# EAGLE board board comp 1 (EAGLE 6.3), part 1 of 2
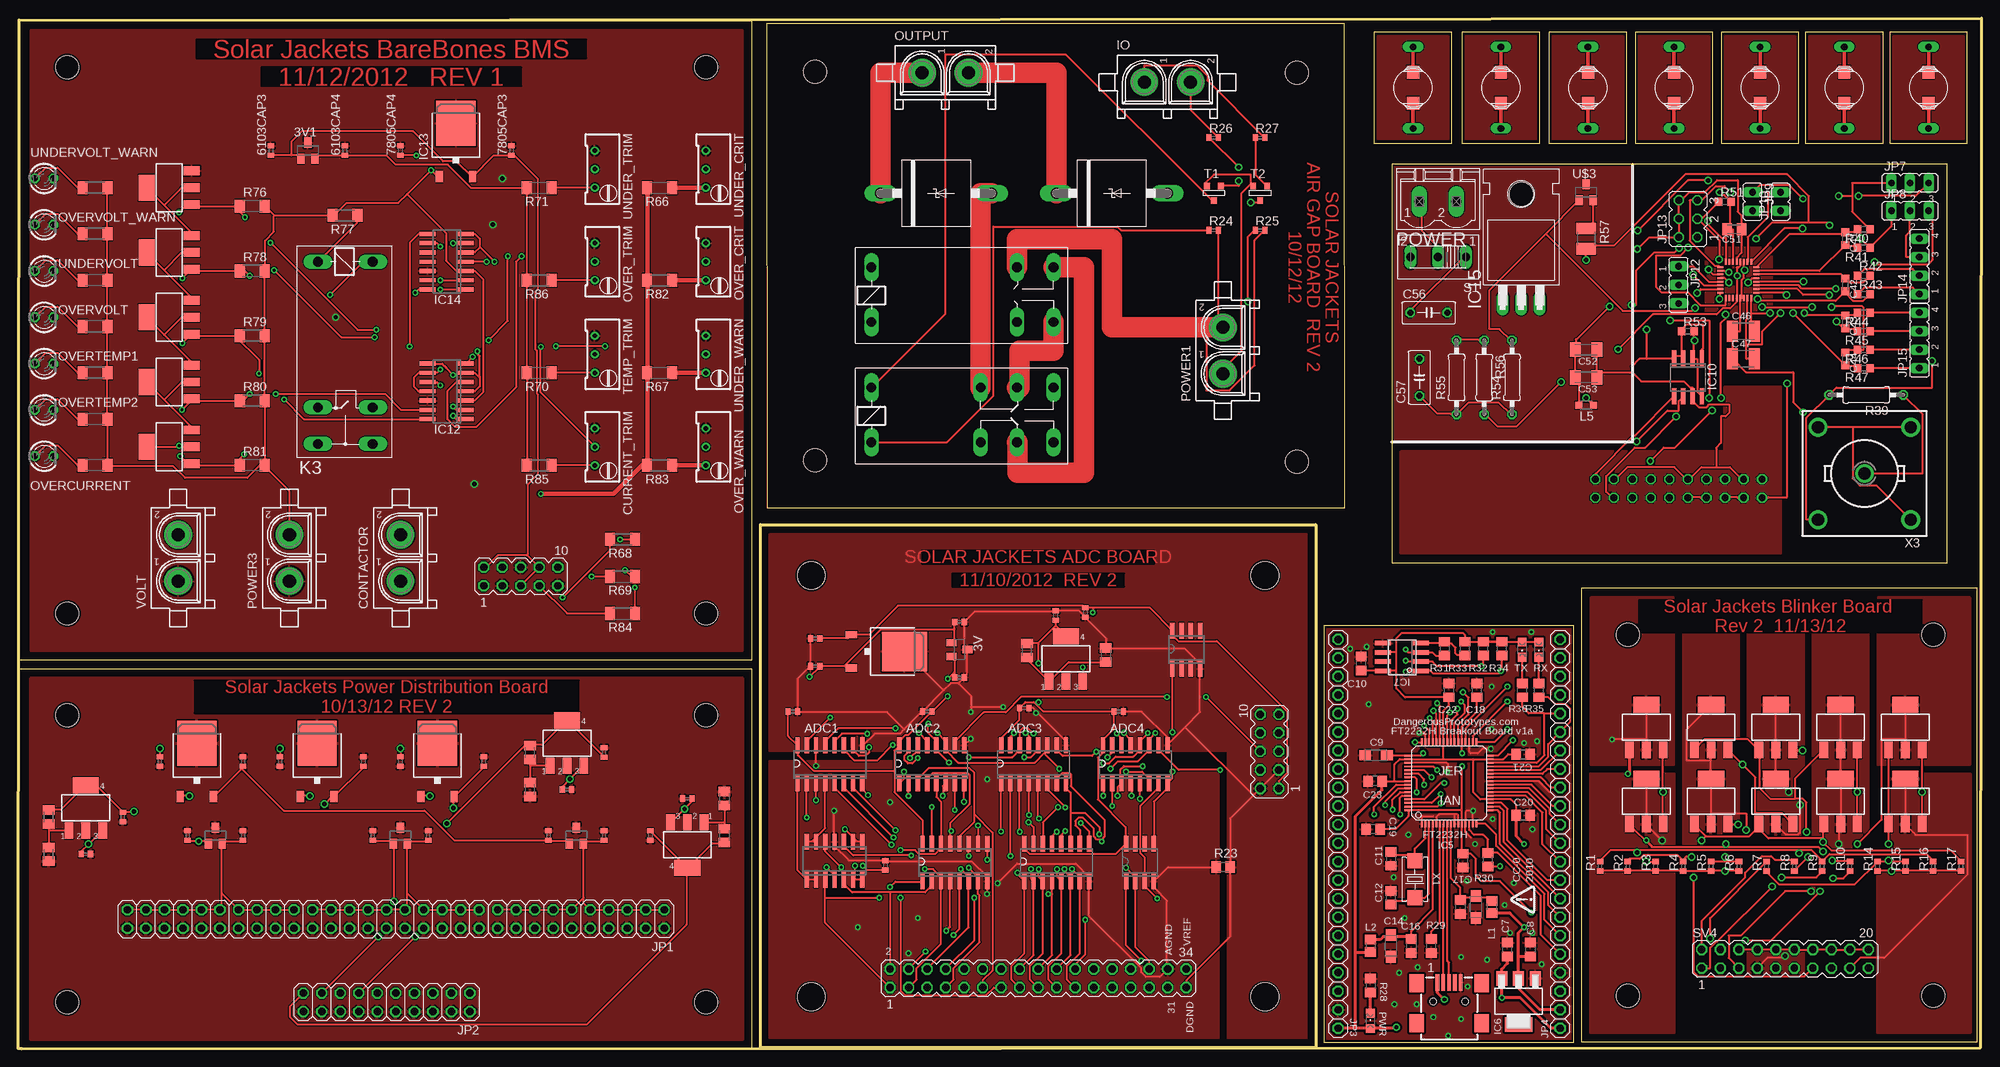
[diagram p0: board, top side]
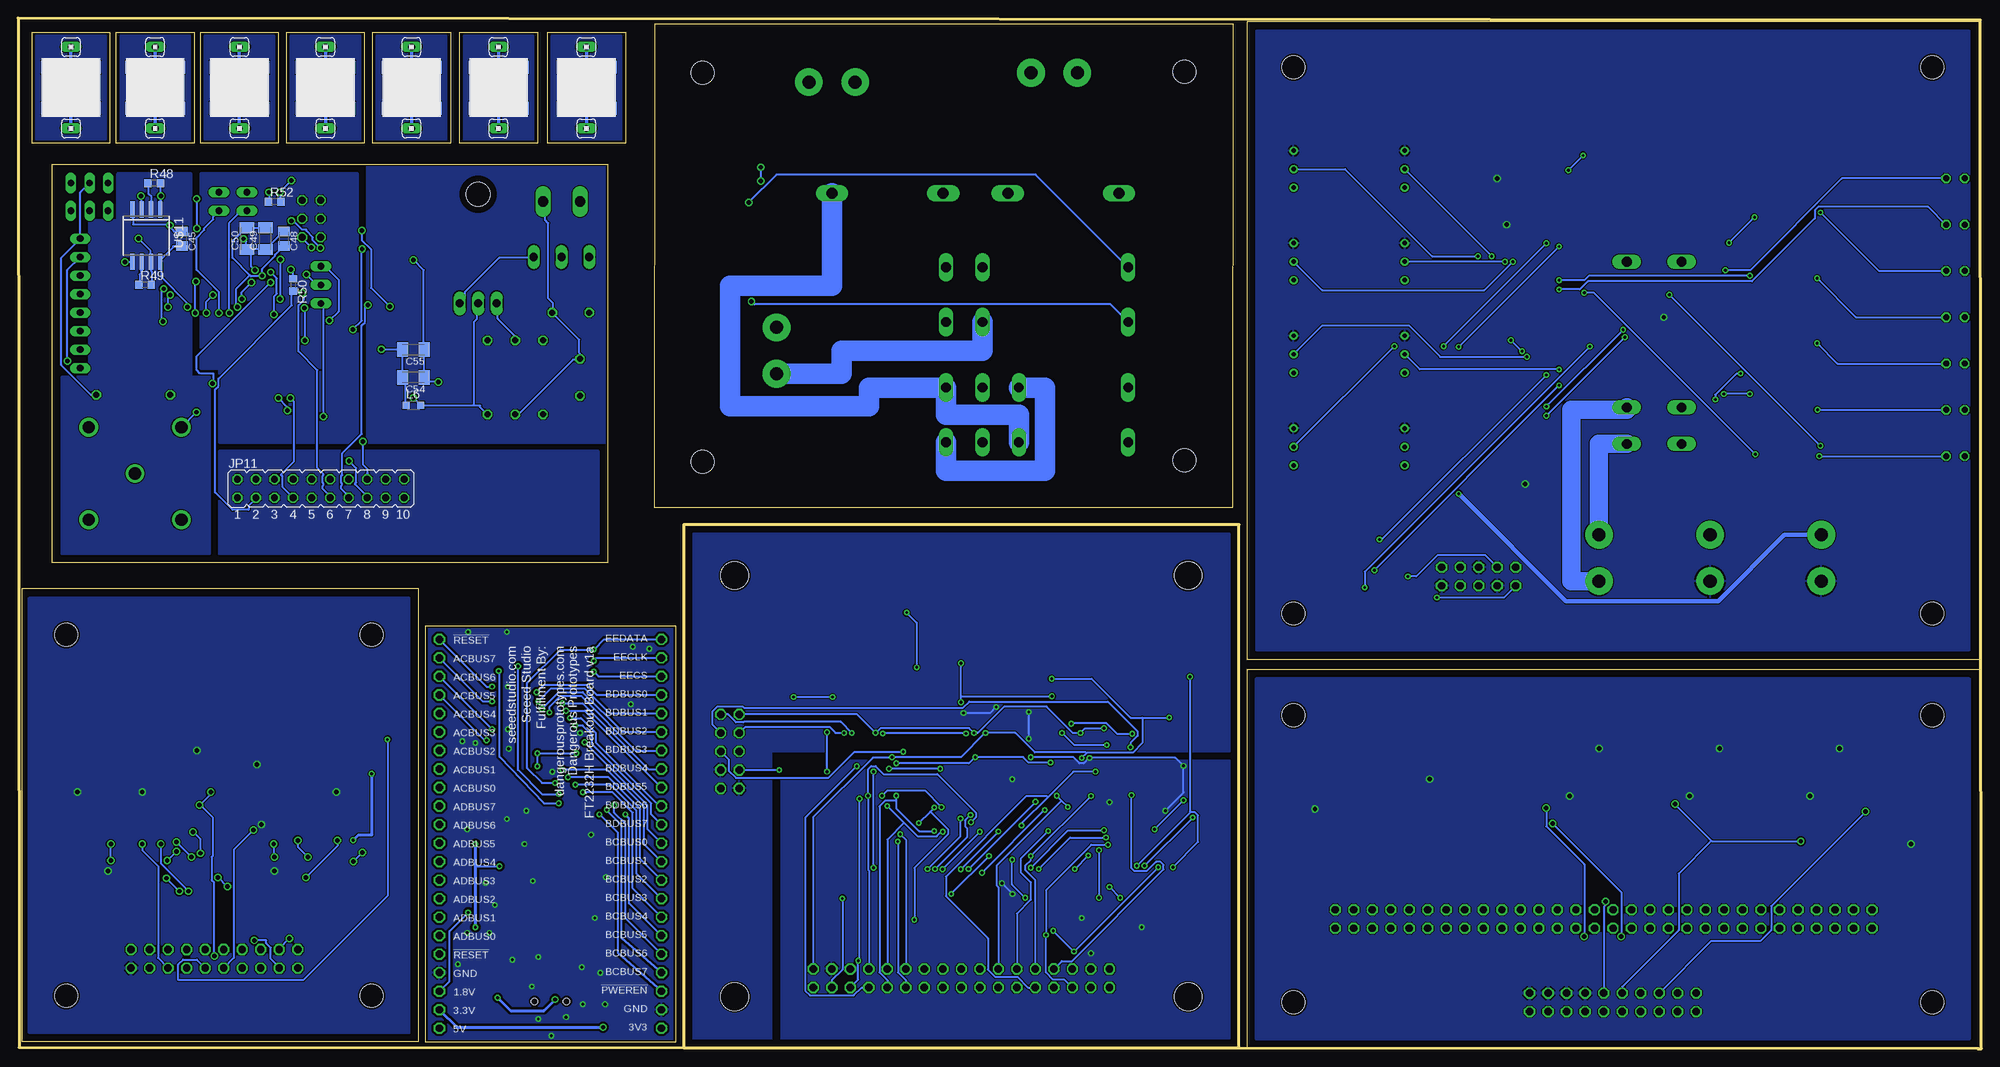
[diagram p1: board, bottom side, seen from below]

Size 269.37 x 141.35 mm. Coordinates in mm from the lower left corner, seen from the top.
Outline: 63 segments
Copper layers (1*16): Top 0.035mm / dielectric 1.5mm / Bottom 0.035mm
Design rules "default *": minimum track width 8mil, minimum drill 15mil, track to track 6mil, track to pad 6mil, pad to pad 6mil, via to via 6mil, smd to smd 6mil, copper to edge 10mil, drill to drill 8mil, minimum pad ring 10mil, minimum via ring 8mil, stop-mask expansion 4mil, vias tented up to drill 0mil, thermal gap 10mil
Holes 3.17 mm at 94.36,59.69 6.73,59.69 94.36,134.62 6.73,134.62 220.85,56.77 220.85,7.24 262.76,56.77 262.76,7.24 94.36,6.35 6.73,6.35 6.73,45.72 94.36,45.72 109.32,80.7 175.48,133.86 175.48,80.52 109.32,134.04
Holes 3.81 mm at 171.07,64.9 108.84,64.9 171.07,7.11 108.84,7.11

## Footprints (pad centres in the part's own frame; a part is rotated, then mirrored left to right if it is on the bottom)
SOT23 = smd 1 x 1.4: 1 -0.95,-1.1; 2 0.95,-1.1; 3 0,1.1
TO252 = smd 1 x 1.6: 1 -2.28,-4.8; 2 2.28,-4.8 | smd 5.4 x 6.2: 3 0,2.5
C0402 = smd 0.7 x 0.9: 1 -0.65,0; 2 0.65,0
SO16 = smd 0.6 x 2.2: 1 -4.445,-2.6; 2 -3.175,-2.6; 3 -1.905,-2.6; 4 -0.635,-2.6; 5 0.635,-2.6; 6 1.905,-2.6; 7 3.175,-2.6; 8 4.445,-2.6; 9 4.445,2.6; 10 3.175,2.6; 11 1.905,2.6; 12 0.635,2.6; 13 -0.635,2.6; 14 -1.905,2.6; 15 -3.175,2.6; 16 -4.445,2.6
SOT223 = smd 1.219 x 2.235: 1 -2.311,-3.099; 2 0,-3.099; 3 2.311,-3.099 | smd 3.6 x 2.2: 4 0,3.099
C805 = smd 1.3 x 1.5: 1 -0.95,0; 2 0.95,0
SMC_A = smd 1.6 x 1.4: + -1.5,0; - 1.5,0
C0603K = smd 1.05 x 1.08: 1 -0.875,0; 2 0.875,0
C0805K = smd 1.3 x 1.6: 1 -1,0; 2 1,0
C1210K = smd 1.5 x 2.9: 1 -1.5,0; 2 1.5,0
C1206K = smd 1.5 x 2: 1 -1.5,0; 2 1.5,0
C050-030X075 = drill 0.813 octagon: 1 -2.54,0; 2 2.54,0
CONN_USB_MINI-B = smd 2 x 2.5: BODY@1 -4.45,2.5; BODY@2 4.45,2.5; BODY@3 4.45,-3; BODY@4 -4.45,-3 | smd 0.5 x 2.3: D+ 0,2.6; D- -0.8,2.6; GND 1.6,2.6; ID 0.8,2.6; VUSB -1.6,2.6 | hole 0.9: -2.2,0; 2.2,0
350428-1 = drill 1.8 pad 3.81: 1 -3.175,0; 2 3.175,0
RTRIM64W = drill 0.61: 1 1.27,-2.54; 2 1.27,0; 3 1.27,2.54
P6T15 = drill 1.499 long: A 7.62,0; C -7.62,0
LQFP64 = smd 1 x 0.27: 1 -5.6,3.75; 2 -5.6,3.25; 3 -5.6,2.75; 4 -5.6,2.25; 5 -5.6,1.75; 6 -5.6,1.25; 7 -5.6,0.75; 8 -5.6,0.25; 9 -5.6,-0.25; 10 -5.6,-0.75; 11 -5.6,-1.25; 12 -5.6,-1.75; 13 -5.6,-2.25; 14 -5.6,-2.75; 15 -5.6,-3.25; 16 -5.6,-3.75; 33 5.6,-3.75; 34 5.6,-3.25; 35 5.6,-2.75; 36 5.6,-2.25; 37 5.6,-1.75; 38 5.6,-1.25; 39 5.6,-0.75; 40 5.6,-0.25; 41 5.6,0.25; 42 5.6,0.75; 43 5.6,1.25; 44 5.6,1.75; 45 5.6,2.25; 46 5.6,2.75; 47 5.6,3.25; 48 5.6,3.75 | smd 0.27 x 1: 17 -3.75,-5.6; 18 -3.25,-5.6; 19 -2.75,-5.6; 20 -2.25,-5.6; 21 -1.75,-5.6; 22 -1.25,-5.6; 23 -0.75,-5.6; 24 -0.25,-5.6; 25 0.25,-5.6; 26 0.75,-5.6; 27 1.25,-5.6; 28 1.75,-5.6; 29 2.25,-5.6; 30 2.75,-5.6; 31 3.25,-5.6; 32 3.75,-5.6; 49 3.75,5.6; 50 3.25,5.6; 51 2.75,5.6; 52 2.25,5.6; 53 1.75,5.6; 54 1.25,5.6; 55 0.75,5.6; 56 0.25,5.6; 57 -0.25,5.6; 58 -0.75,5.6; 59 -1.25,5.6; 60 -1.75,5.6; 61 -2.25,5.6; 62 -2.75,5.6; 63 -3.25,5.6; 64 -3.75,5.6
SOT223' = smd 1.5 x 2: 1 -2.3,-3.15; 2 0,-3.15; 3 2.3,-3.15 | smd 3.8 x 2: 4 0,3.15
SOIC8 = smd 0.6 x 2.2: 1 -1.905,-2.6; 2 -0.635,-2.6; 3 0.635,-2.6; 4 1.905,-2.6; 5 1.905,2.6; 6 0.635,2.6; 7 -0.635,2.6; 8 -1.905,2.6
SO-08 = smd 0.6 x 2.2: 1 -1.905,-2.6; 2 -0.635,-2.6; 3 0.635,-2.6; 4 1.905,-2.6; 5 1.905,2.6; 6 0.635,2.6; 7 -0.635,2.6; 8 -1.905,2.6
SO14 = smd 0.6 x 2.2: 1 -3.81,-2.6; 2 -2.54,-2.6; 3 -1.27,-2.6; 4 0,-2.6; 5 1.27,-2.6; 6 2.54,-2.6; 7 3.81,-2.6; 8 3.81,2.6; 9 2.54,2.6; 10 1.27,2.6; 11 0,2.6; 12 -1.27,2.6; 13 -2.54,2.6; 14 -3.81,2.6
TO220H = drill 1.118 long: 1 -2.54,-10.16; 2 0,-10.16; 3 2.54,-10.16 | hole 3.302: 0,4.826
2X30 = drill 1.016 octagon: 1 -38.1,-1.27; 2 -38.1,1.27; 3 -35.56,-1.27; 4 -35.56,1.27; 5 -33.02,-1.27; 6 -33.02,1.27; 7 -30.48,-1.27; 8 -30.48,1.27; 9 -27.94,-1.27; 10 -27.94,1.27; 11 -25.4,-1.27; 12 -25.4,1.27; 13 -22.86,-1.27; 14 -22.86,1.27; 15 -20.32,-1.27; 16 -20.32,1.27; 17 -17.78,-1.27; 18 -17.78,1.27; 19 -15.24,-1.27; 20 -15.24,1.27; 21 -12.7,-1.27; 22 -12.7,1.27; 23 -10.16,-1.27; 24 -10.16,1.27; 25 -7.62,-1.27; 26 -7.62,1.27; 27 -5.08,-1.27; 28 -5.08,1.27; 29 -2.54,-1.27; 30 -2.54,1.27; 31 0,-1.27; 32 0,1.27; 33 2.54,-1.27; 34 2.54,1.27; 35 5.08,-1.27; 36 5.08,1.27; 37 7.62,-1.27; 38 7.62,1.27; 39 10.16,-1.27; 40 10.16,1.27; 41 12.7,-1.27; 42 12.7,1.27; 43 15.24,-1.27; 44 15.24,1.27; 45 17.78,-1.27; 46 17.78,1.27; 47 20.32,-1.27; 48 20.32,1.27; 49 22.86,-1.27; 50 22.86,1.27; 51 25.4,-1.27; 52 25.4,1.27; 53 27.94,-1.27; 54 27.94,1.27; 55 30.48,-1.27; 56 30.48,1.27; 57 33.02,-1.27; 58 33.02,1.27; 59 35.56,-1.27; 60 35.56,1.27
2X10 = drill 1.016 octagon: 1 -11.43,-1.27; 2 -11.43,1.27; 3 -8.89,-1.27; 4 -8.89,1.27; 5 -6.35,-1.27; 6 -6.35,1.27; 7 -3.81,-1.27; 8 -3.81,1.27; 9 -1.27,-1.27; 10 -1.27,1.27; 11 1.27,-1.27; 12 1.27,1.27; 13 3.81,-1.27; 14 3.81,1.27; 15 6.35,-1.27; 16 6.35,1.27; 17 8.89,-1.27; 18 8.89,1.27; 19 11.43,-1.27; 20 11.43,1.27
1X22 = drill 1.016 octagon: 1 -26.67,0; 2 -24.13,0; 3 -21.59,0; 4 -19.05,0; 5 -16.51,0; 6 -13.97,0; 7 -11.43,0; 8 -8.89,0; 9 -6.35,0; 10 -3.81,0; 11 -1.27,0; 12 1.27,0; 13 3.81,0; 14 6.35,0; 15 8.89,0; 16 11.43,0; 17 13.97,0; 18 16.51,0; 19 19.05,0; 20 21.59,0; 21 24.13,0; 22 26.67,0
JP2 = drill 0.914 long: 1 -2.54,0; 2 0,0; 3 2.54,0
JP1 = drill 0.914 long: 1 0,-1.27; 2 0,1.27
JP10Q = drill 0.914 octagon: 1 -11.43,-1.27; 2 -11.43,1.27; 3 -8.89,-1.27; 4 -8.89,1.27; 5 -6.35,-1.27; 6 -6.35,1.27; 7 -3.81,-1.27; 8 -3.81,1.27; 9 -1.27,-1.27; 10 -1.27,1.27; 11 1.27,-1.27; 12 1.27,1.27; 13 3.81,-1.27; 14 3.81,1.27; 15 6.35,-1.27; 16 6.35,1.27; 17 8.89,-1.27; 18 8.89,1.27; 19 11.43,-1.27; 20 11.43,1.27
JP3Q = drill 0.914 octagon: 1 -2.54,-1.27; 2 -2.54,1.27; 3 0,-1.27; 4 0,1.27; 5 2.54,-1.27; 6 2.54,1.27
JP4 = drill 0.914 long: 1 -3.81,0; 2 -1.27,0; 3 1.27,0; 4 3.81,0
G2R2 = drill 1.321 long: 1 -2.54,-3.683; 2 -2.54,3.81; O1 12.471,3.81; O2 12.471,-3.683; P1 17.45,3.81; P2 17.45,-3.683; S1 22.454,3.81; S2 22.454,-3.683
G2R2A = drill 1.321 long: 1 -2.54,-3.683; 2 -2.54,3.81; P1 17.45,3.81; P2 17.45,-3.683; S1 22.454,3.81; S2 22.454,-3.683
G2REA = drill 1.321 long: 1 -2.54,-3.683; 2 -2.54,3.81; P 17.45,-3.683; P@ 17.45,3.81; S 22.454,-3.683; S@ 22.454,3.81
FB805 = smd 1.3 x 1.5: 1 -0.85,0; 2 0.85,0
L2012C = smd 1 x 1: 1 -1,0; 2 1,0
LQH55PN220MR0L = smd 1.8 x 1.7: P$1 -2.135,0; P$2 2.135,0
NRS8040T0R9NJGJ = smd 8.2 x 1.8: P$1 0,2.8; P$2 0,-2.8
LED3MM = drill 0.813 octagon: A -1.27,0; K 1.27,0
MSTBV2 = drill 1.397 long: 1 -2.54,0; 2 2.54,0
LED-805 = smd 1.2 x 1.2: A 0,-1.05; C 0,1.05
R0402 = smd 0.7 x 0.9: 1 -0.65,0; 2 0.65,0
M0805 = smd 1.3 x 1.6: 1 -0.95,0; 2 0.95,0
R805 = smd 1.3 x 1.5: 1 -0.95,0; 2 0.95,0
0207/10 = drill 0.813 octagon: 1 -5.08,0; 2 5.08,0
R0603 = smd 1 x 1.1: 1 -0.85,0; 2 0.85,0
R3225 = smd 1.6 x 2.7: 1 -1.4,0; 2 1.4,0
M1406 = smd 1.4 x 1.8: 1 -1.7,0; 2 1.7,0
255SB = drill 1.118 long: 1 -3.81,0; 2 0,0; 3 3.81,0
MA17-2 = drill 1.016 octagon: 1 -20.32,-1.27; 2 -20.32,1.27; 3 -17.78,-1.27; 4 -17.78,1.27; 5 -15.24,-1.27; 6 -15.24,1.27; 7 -12.7,-1.27; 8 -12.7,1.27; 9 -10.16,-1.27; 10 -10.16,1.27; 11 -7.62,-1.27; 12 -7.62,1.27; 13 -5.08,-1.27; 14 -5.08,1.27; 15 -2.54,-1.27; 16 -2.54,1.27; 17 0,-1.27; 18 0,1.27; 19 2.54,-1.27; 20 2.54,1.27; 21 5.08,-1.27; 22 5.08,1.27; 23 7.62,-1.27; 24 7.62,1.27; 25 10.16,-1.27; 26 10.16,1.27; 27 12.7,-1.27; 28 12.7,1.27; 29 15.24,-1.27; 30 15.24,1.27; 31 17.78,-1.27; 32 17.78,1.27; 33 20.32,-1.27; 34 20.32,1.27
MA05-2 = drill 1.016 octagon: 1 -5.08,-1.27; 2 -5.08,1.27; 3 -2.54,-1.27; 4 -2.54,1.27; 5 0,-1.27; 6 0,1.27; 7 2.54,-1.27; 8 2.54,1.27; 9 5.08,-1.27; 10 5.08,1.27
MA10-2 = drill 1.016 octagon: 1 -11.43,-1.27; 2 -11.43,1.27; 3 -8.89,-1.27; 4 -8.89,1.27; 5 -6.35,-1.27; 6 -6.35,1.27; 7 -3.81,-1.27; 8 -3.81,1.27; 9 -1.27,-1.27; 10 -1.27,1.27; 11 1.27,-1.27; 12 1.27,1.27; 13 3.81,-1.27; 14 3.81,1.27; 15 6.35,-1.27; 16 6.35,1.27; 17 8.89,-1.27; 18 8.89,1.27; 19 11.43,-1.27; 20 11.43,1.27
SOT-23 = smd 0.787 x 0.889: 1 0.025,-1.016; 2 -0.94,1.016; 3 0.991,1.016
ADS8363 = smd 0.28 x 0.85: P$1_ 0.725,0.725; P$2_ 1.225,0.725; P$3_ 1.725,0.725; P$4_ 2.225,0.725; P$5_ 2.725,0.725; P$6_ 3.225,0.725; P$7_ 3.725,0.725; P$8_ 4.225,0.725; P$17_ 4.225,-4.225; P$18_ 3.725,-4.225; P$19_ 3.225,-4.225; P$20_ 2.725,-4.225; P$21_ 2.225,-4.225; P$22_ 1.725,-4.225; P$23_ 1.225,-4.225; P$24_ 0.725,-4.225 | smd 0.85 x 0.28: P$9_ 4.95,0; P$10_ 4.95,-0.5; P$11_ 4.95,-1; P$12_ 4.95,-1.5; P$13_ 4.95,-2; P$14_ 4.95,-2.5; P$15_ 4.95,-3; P$16_ 4.95,-3.5; P$25_ 0,-3.5; P$26_ 0,-3; P$27_ 0,-2.5; P$28_ 0,-2; P$29_ 0,-1.5; P$30_ 0,-1; P$31_ 0,-0.5; P$32_ 0,0
SINGLE_HEADER = drill 0.914 long: P$1 0,0
SOP-08 = smd 0.6 x 2.2: 1 -1.905,-3.6; 2 -0.635,-3.6; 3 0.635,-3.6; 4 1.905,-3.6; 5 1.905,3.575; 6 0.635,3.575; 7 -0.635,3.575; 8 -1.905,3.575
4X6 = smd 2.032 x 2.032: 1 -2.54,0; 2 2.54,0
B35N57 = drill 1.7: 1 0,0; 2 6.35,6.35; 3 -6.35,6.35; 4 -6.35,-6.35; 5 6.35,-6.35

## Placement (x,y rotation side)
3V  MAX6103  [SOT23]  129.16,54.74 270 top
3V1  MAX6103  [SOT23]  39.75,123.19 0 top
3V2  MAX6103  [SOT23]  76.58,29.21 0 top
3V3  MAX6103  [SOT23]  52.45,29.21 0 top
3V4  MAX6103  [SOT23]  27.05,29.21 0 top
5V  LM7805TV  [TO252]  119.13,54.48 270 top
317CAP1  .33uF  [C0402]  146.43,59.82 270 top
317CAP2  1uF  [C0402]  142.37,59.44 90 top
317CAP3  .33uF  [C0402]  9.27,26.67 0 top
317CAP4  1uF  [C0402]  14.35,31.75 270 top
317CAP5  .33uF  [C0402]  75.31,35.56 0 top
317CAP6  1uF  [C0402]  80.39,40.64 90 top
317CAP7  .33uF  [C0402]  91.82,34.29 180 top
317CAP8  1uF  [C0402]  86.74,29.21 270 top
6103CAP1  1uF  [C0402]  129.16,58.55 0 top
6103CAP2  1uF  [C0402]  129.16,50.93 0 top
6103CAP3  1uF  [C0402]  34.67,123.19 90 top
6103CAP4  1uF  [C0402]  44.83,123.19 90 top
6103CAP5  1uF  [C0402]  72.77,29.21 90 top
6103CAP6  1uF  [C0402]  80.39,29.21 90 top
6103CAP7  1uF  [C0402]  48.64,29.21 90 top
6103CAP8  1uF  [C0402]  56.26,29.21 90 top
6103CAP9  1uF  [C0402]  23.24,29.21 90 top
6103CAP10  1uF  [C0402]  30.86,29.21 90 top
6484CAP1  .1uF  [C0402]  119,25.15 90 top
7805CAP1  .33uF  [C0402]  109.35,56.26 180 top
7805CAP2  1uF  [C0402]  109.35,52.45 180 top
7805CAP3  1uF  [C0402]  67.69,123.19 90 top
7805CAP4  1uF  [C0402]  52.45,123.19 90 top
ADC1  MCP-3008  [SO16]  111.38,38.99 0 top
ADC2  MCP-3008  [SO16]  125.35,38.99 0 top
ADC3  MCP-3008  [SO16]  139.32,38.99 0 top
ADC4  MCP-3008  [SO16]  153.29,38.99 0 top
ADC_CAP1  .1uF  [C0402]  106.3,46.23 0 top
ADC_CAP2  .1uF  [C0402]  124.71,46.23 180 top
ADC_CAP3  .1uF  [C0402]  138.05,46.74 0 top
ADC_CAP4  .1uF  [C0402]  151,46.23 0 top
BLINKER-L1  N-HEXFET-2D_SOT232-  [SOT223]  223.39,44.07 0 top
BLINKER-L2  N-HEXFET-2D_SOT232-  [SOT223]  223.39,33.91 0 top
BLINKER-R1  N-HEXFET-2D_SOT232-  [SOT223]  258.95,44.07 0 top
BLINKER-R2  N-HEXFET-2D_SOT232-  [SOT223]  258.95,33.91 0 top
BRAKE-C1  N-HEXFET-2D_SOT232-  [SOT223]  241.17,44.07 0 top
BRAKE-C2  N-HEXFET-2D_SOT232-  [SOT223]  241.17,33.91 0 top
BRAKE-L1  N-HEXFET-2D_SOT232-  [SOT223]  232.28,44.07 0 top
BRAKE-L2  N-HEXFET-2D_SOT232-  [SOT223]  232.28,33.91 0 top
BRAKE-R1  N-HEXFET-2D_SOT232-  [SOT223]  250.06,44.07 0 top
BRAKE-R2  N-HEXFET-2D_SOT232-  [SOT223]  250.06,33.91 0 top
C1  1uF  [C0402]  19.43,39.37 270 top
C2  1uF  [C0402]  30.86,39.37 90 top
C3  1uF  [C0402]  35.94,39.37 270 top
C4  1uF  [C0402]  47.37,39.37 90 top
C5  1uF  [C0402]  52.45,39.37 270 top
C6  1uF  [C0402]  63.88,39.37 90 top
C7  0.1uF  [C805]  204.34,13.59 90 top
C8  0.1uF  [C805]  207.52,13.59 90 top
C9  3.3uF  [SMC_A]  186.31,40.26 180 top
C10  0.1uF  [C805]  184.28,52.83 90 top
C11  27pF  [C805]  188.34,26.04 270 top
C12  27pF  [C805]  188.34,20.7 90 top
C13  4.7uF  [SMC_A]  200.03,19.43 270 top
C14  4.7uF  [SMC_A]  188.34,14.1 270 top
C15  0.1uF  [C805]  197.87,19.43 270 top
C16  0.1uF  [C805]  191.13,14.1 270 top
C17  0.1uF  [C805]  198.25,25.78 270 top
C18  0.1uF  [C805]  200.15,49.15 90 top
C19  0.1uF  [C805]  185.93,30.1 180 top
C20  0.1uF  [C805]  206.5,32 0 top
C21  0.1uF  [C805]  206.5,40.39 0 top
C22  0.1uF  [C805]  196.34,49.15 90 top
C23  0.1uF  [C805]  186.18,36.7 180 top
C41  3900pF  [C0603K]  250.7,111.12 270 top
C42  3900pF  [C0603K]  250.7,104.78 270 top
C43  3900pF  [C0603K]  250.7,99.69 270 top
C44  3900pF  [C0603K]  250.7,94.61 270 top
C45  1uF  [C0805K]  246.89,111.12 270 bottom
C46  10uF  [C1210K]  236.73,98.42 0 top
C47  10uF  [C1210K]  236.73,94.61 0 top
C48  1uF  [C0805K]  232.92,111.12 270 bottom
C49  0.1uF  [C1206K]  235.46,111.12 90 bottom
C50  0.1uF  [C1206K]  238,111.12 90 bottom
C51  1uF  [C0805K]  235.46,112.39 180 top
C52  0.1uF  [C1206K]  215.14,95.89 180 top
C53  0.1uF  [C1206K]  215.14,92.08 180 top
C54  0.1uF  [C1206K]  215.14,92.08 180 bottom
C55  0.1uF  [C1206K]  215.14,95.89 180 bottom
C56  [C050-030X075]  193.55,100.97 0 top
C57  [C050-030X075]  192.28,92.08 90 top
CONN1  CONN_USB  [CONN_USB_MINI-B]  196.34,6.48 0 top
CONTACTOR  350428-1  [350428-1]  52.45,67.31 90 top
CURRENT_TRIM  1k  [RTRIM64W]  80.39,82.55 180 top
D1  5KPXX  [P6T15]  125.95,117.35 0 top
D2  5KPXX  [P6T15]  150.08,117.35 0 top
IC1  LM317  [SOT223]  75.31,41.91 0 top
IC2  LM317  [SOT223]  9.27,33.02 0 top
IC3  LM317  [SOT223]  91.82,27.94 180 top
IC4  LM317  [SOT223]  143.76,53.47 0 top
IC5  FT2232H  [LQFP64]  196.34,36.45 90 top
IC6  [SOT223']  205.87,6.48 180 top
IC7  93C46  [SOIC8]  189.87,53.72 90 top
IC10  24LC256T  [SO-08]  229.11,92.08 180 top
IC12  LM339D  [SO14]  58.8,90.17 90 top
IC13  7805DT  [TO252]  60.07,124.46 0 top
IC14  LM339D  [SO14]  58.8,107.95 90 top
IC15  317T  [TO220H]  206.25,112.39 0 top
IO  350428-1  [350428-1]  157.7,132.59 0 top
JP1  [2X30]  50.55,17.78 180 top
JP2  [2X10]  50.55,6.35 180 top
JP3  [1X22]  181.1,29.46 90 top
JP4  [1X22]  211.58,29.46 90 top
JP7  [JP2]  259.59,118.75 0 top
JP8  [JP2]  259.59,114.94 0 top
JP9  [JP1]  238,116.2 180 top
JP10  [JP1]  241.81,116.2 0 top
JP11  [JP10Q]  227.84,76.83 0 bottom
JP12  [JP2]  227.84,104.78 270 top
JP13  [JP3Q]  229.13,113.84 90 top
JP14  [JP4]  260.86,107.31 90 top
JP15  [JP4]  260.86,97.16 90 top
K1  G2R2  [G2R2]  119.6,86.87 0 top
K2  G2R2A  [G2R2A]  119.6,103.38 0 top
K3  G2REA  [G2REA]  44.83,105.41 270 top
L1  [FB805]  202.18,19.43 270 top
L2  [FB805]  185.55,14.1 270 top
L5  [L2012C]  215.14,88.27 180 top
L6  [L2012C]  215.14,88.27 0 bottom
LMC6484_1  LMC6484  [SO14]  112.01,25.78 0 top
NEWBATT  LQH55PN220MR0L  [LQH55PN220MR0L]  191.39,131.83 270 top
NEWBATT1  LQH55PN220MR0L  [LQH55PN220MR0L]  203.45,131.83 270 top
NEWBATT2  LQH55PN220MR0L  [LQH55PN220MR0L]  215.39,131.83 270 top
NEWBATT3  LQH55PN220MR0L  [LQH55PN220MR0L]  227.2,131.83 270 top
NEWBATT4  LQH55PN220MR0L  [LQH55PN220MR0L]  239.01,131.83 270 top
NEWBATT5  LQH55PN220MR0L  [LQH55PN220MR0L]  250.57,131.83 270 top
NEWBATT6  LQH55PN220MR0L  [LQH55PN220MR0L]  262.13,131.83 270 top
OLDBATT  NRS8040T0R9NJGJ  [NRS8040T0R9NJGJ]  191.39,131.83 0 bottom
OLDBATT1  NRS8040T0R9NJGJ  [NRS8040T0R9NJGJ]  203.45,131.83 0 bottom
OLDBATT2  NRS8040T0R9NJGJ  [NRS8040T0R9NJGJ]  215.39,131.83 0 bottom
OLDBATT3  NRS8040T0R9NJGJ  [NRS8040T0R9NJGJ]  227.2,131.83 0 bottom
OLDBATT4  NRS8040T0R9NJGJ  [NRS8040T0R9NJGJ]  239.01,131.83 0 bottom
OLDBATT5  NRS8040T0R9NJGJ  [NRS8040T0R9NJGJ]  250.57,131.83 0 bottom
OLDBATT6  NRS8040T0R9NJGJ  [NRS8040T0R9NJGJ]  262.13,131.83 0 bottom
OUTPUT  350428-1  [350428-1]  127.22,133.86 0 top
OVER_CRIT  10k  [RTRIM64W]  95.63,107.95 180 top
OVER_TRIM  1k  [RTRIM64W]  80.39,107.95 180 top
OVER_WARN  10K  [RTRIM64W]  95.63,82.55 180 top
OVERCURRENT  TLLG4400  [LED3MM]  3.56,81.28 0 top
OVERCURRENT_FET  N-HEXFET-2D_SOT232-  [SOT223]  20.7,82.55 90 top
OVERTEMP1  TLLG4400  [LED3MM]  3.56,93.98 0 top
OVERTEMP1_FET  N-HEXFET-2D_SOT232-  [SOT223]  20.7,100.33 90 top
OVERTEMP2  TLLG4400  [LED3MM]  3.56,87.63 0 top
OVERTEMP2_FET  N-HEXFET-2D_SOT232-  [SOT223]  20.7,91.44 90 top
OVERVOLT  TLLG4400  [LED3MM]  3.56,100.33 0 top
OVERVOLT_FET  N-HEXFET-2D_SOT232-  [SOT223]  20.7,109.22 90 top
OVERVOLT_WARN  TLLG4400  [LED3MM]  3.56,113.03 0 top
POWER  MSTBV2  [MSTBV2]  194.82,116.2 0 top
POWER1  350428-1  [350428-1]  165.32,95.76 90 top
POWER3  350428-1  [350428-1]  37.21,67.31 90 top
PWR  [LED-805]  185.55,3.81 0 top
PWR_1  7805DT  [TO252]  24.51,39.37 0 top
PWR_2  7805DT  [TO252]  41.02,39.37 0 top
PWR_3  7805DT  [TO252]  57.53,39.37 0 top
R1  1k  [R0402]  217.04,25.02 90 top
R2  1k  [R0402]  220.85,25.02 90 top
R3  1k  [R0402]  224.66,25.02 90 top
R4  1k  [R0402]  228.47,25.02 90 top
R5  1k  [R0402]  232.28,25.02 90 top
R6  1k  [R0402]  236.09,25.02 90 top
R7  1K  [R0402]  239.9,25.02 90 top
R8  1K  [R0402]  243.71,25.02 90 top
R9  1K  [R0402]  247.52,25.02 90 top
R10  1K  [R0402]  251.33,25.02 90 top
R11  220  [M0805]  4.19,31.75 270 top
R12  361  [M0805]  4.19,26.67 270 top
R13  220  [M0805]  70.23,40.64 270 top
R14  1k  [R0402]  255.14,25.02 90 top
R15  1k  [R0402]  258.95,25.02 90 top
R16  1k  [R0402]  262.76,25.02 90 top
R17  1k  [R0402]  266.57,25.02 90 top
R18  361  [M0805]  70.23,35.56 270 top
R19  220  [M0805]  96.9,29.21 90 top
R20  361  [M0805]  96.9,34.29 90 top
R21  220  [M0805]  138.43,54.61 270 top
R22  361  [M0805]  149.22,53.98 90 top
R23  0  [M0805]  165.35,24.89 0 top
R24  1k  [R0402]  164.05,112.27 0 top
R25  1k  [R0402]  170.4,112.27 0 top
R26  1k  [R0402]  164.05,124.97 0 top
R27  1k  [R0402]  170.4,124.97 0 top
R28  470  [R805]  185.55,8.64 270 top
R29  12k 1%  [R805]  193.93,14.1 90 top
R30  10k  [R805]  201.68,25.91 90 top
R31  2.2k  [R805]  195.71,54.86 270 top
R32  10k  [R805]  201.04,54.86 90 top
R33  10k  [R805]  198.5,54.86 90 top
R34  10k  [R805]  203.58,54.86 90 top
R35  470  [R805]  208.66,49.15 90 top
R36  470  [R805]  206.38,49.15 90 top
R39  1M  [0207/10]  253.57,89.69 180 top
R40  49.9  [R0603]  253.24,112.39 180 top
R41  49.9  [R0603]  253.24,109.86 180 top
R42  49.9  [R0603]  253.24,106.05 0 top
R43  49.9  [R0603]  253.24,103.5 0 top
R44  49.9  [R0603]  253.24,100.97 180 top
R45  49.9  [R0603]  253.24,98.42 180 top
R46  49.9  [R0603]  253.24,95.89 180 top
R47  49.9  [R0603]  253.24,93.34 180 top
R48  49.9  [R0603]  250.7,118.75 0 bottom
R49  49.9  [R0603]  251.97,104.78 0 bottom
R50  33  [R0603]  231.65,104.78 270 bottom
R51  10K  [R0603]  234.19,116.2 0 top
R52  10K  [R0603]  234.19,116.2 0 bottom
R53  33  [R0603]  229.11,98.42 0 top
R54  150  [0207/10]  204.98,92.08 90 top
R55  240  [0207/10]  197.36,92.08 90 top
R56  725  [0207/10]  201.17,92.08 270 top
R57  0  [R3225]  215.14,111.12 270 top
R66  100k  [M1406]  88.01,118.11 180 top
R67  100k  [M1406]  88.01,92.71 180 top
R68  100  [M1406]  82.93,69.85 180 top
R69  100  [M1406]  82.93,64.77 180 top
R70  100  [M1406]  71.5,92.71 180 top
R71  100  [M1406]  71.5,118.11 180 top
R72  1k  [M1406]  10.54,105.41 0 top
R73  1k  [M1406]  10.54,118.11 0 top
R74  1k  [M1406]  10.54,92.71 0 top
R75  1k  [M1406]  10.54,86.36 0 top
R76  1k  [M1406]  32.13,115.57 0 top
R77  100  [M1406]  44.83,114.3 180 top
R78  1k  [M1406]  32.13,106.68 0 top
R79  1k  [M1406]  32.13,97.79 0 top
R80  1k  [M1406]  32.13,88.9 0 top
R81  1k  [M1406]  32.13,80.01 0 top
R82  100k  [M1406]  88.01,105.41 180 top
R83  100k  [M1406]  88.01,80.01 180 top
R84  1k  [M1406]  82.93,59.69 180 top
R85  100  [M1406]  71.5,80.01 180 top
R86  100  [M1406]  71.5,105.41 180 top
R87  1k  [M1406]  10.54,99.06 0 top
R88  1k  [M1406]  10.54,111.76 0 top
R89  1k  [M1406]  10.54,80.01 0 top
RX  [LED-805]  208.66,54.74 180 top
S1  [255SB]  194.82,108.58 180 top
SV1  [MA17-2]  139.95,9.65 0 top
SV2  [MA05-2]  171.7,40.77 90 top
SV3  [MA05-2]  68.96,64.77 0 top
SV4  [MA10-2]  242.44,12.32 0 top
T1  [SOT-23]  164.05,117.35 0 top
T2  [SOT-23]  170.4,117.35 0 top
TEMP_TRIM  1k  [RTRIM64W]  80.39,95.25 180 top
TX  [LED-805]  206.38,54.74 180 top
U$1  LM35  [SO-08]  160.27,54.74 0 top
U$2  ADS8386  [ADS8363]  237.79,107.93 270 top
U$3  LM4040  [SOT23]  215.14,117.47 0 top
U$4  [DP_LOGO]  207.52,20.45 90 top
U$5  SINGLE_HEADER  [SINGLE_HEADER]  191.39,126.24 0 bottom
U$6  SP720APP  [SO16]  128.52,25.53 0 top
U$7  SP720APP  [SO16]  142.49,25.53 0 top
U$8  SP721APP  [SO-08]  153.92,25.53 0 top
U$9  SINGLE_HEADER  [SINGLE_HEADER]  191.39,137.41 180 bottom
U$10  SINGLE_HEADER  [SINGLE_HEADER]  203.45,126.24 0 bottom
U$11  OPA2365  [SOP-08]  251.79,111.51 180 bottom
U$12  SINGLE_HEADER  [SINGLE_HEADER]  203.45,137.41 180 bottom
U$13  SINGLE_HEADER  [SINGLE_HEADER]  215.39,126.24 0 bottom
U$14  SINGLE_HEADER  [SINGLE_HEADER]  215.39,137.41 180 bottom
U$15  SINGLE_HEADER  [SINGLE_HEADER]  227.2,126.24 0 bottom
U$16  SINGLE_HEADER  [SINGLE_HEADER]  227.2,137.41 180 bottom
U$17  SINGLE_HEADER  [SINGLE_HEADER]  239.01,126.24 0 bottom
U$18  SINGLE_HEADER  [SINGLE_HEADER]  239.01,137.41 180 bottom
U$19  SINGLE_HEADER  [SINGLE_HEADER]  250.57,126.24 0 bottom
U$20  SINGLE_HEADER  [SINGLE_HEADER]  250.57,137.41 180 bottom
U$21  SINGLE_HEADER  [SINGLE_HEADER]  262.13,126.24 0 bottom
U$22  SINGLE_HEADER  [SINGLE_HEADER]  262.13,137.41 180 bottom
UNDER_CRIT  10k  [RTRIM64W]  95.63,120.65 180 top
UNDER_TRIM  1k  [RTRIM64W]  80.39,120.65 180 top
UNDER_WARN  10K  [RTRIM64W]  95.63,95.25 180 top
UNDERVOLT  TLLG4400  [LED3MM]  3.56,106.68 0 top
UNDERVOLT_FET  N-HEXFET-2D_SOT232-  [SOT223]  20.7,118.11 90 top
UNDERVOLT_WARN  TLLG4400  [LED3MM]  3.56,119.38 0 top
VOLT  350428-1  [350428-1]  21.97,67.31 90 top
X1  12MHz  [4X6]  191.64,23.24 270 top
X3  B35N57  [B35N57]  253.34,78.89 180 top

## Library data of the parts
3V 3V1-3V4 ADC1-ADC4 LMC6484_1 U$1 U$6-U$8 = SolarJacketsADC
5V IC1-IC4 IC12-IC15 PWR_1-PWR_3 = linear
317CAP1-317CAP8 6103CAP1-6103CAP10 6484CAP1 7805CAP1-7805CAP4 ADC_CAP1-ADC_CAP4 C1-C6 C41-C55 CURRENT_TRIM OVER_CRIT OVER_TRIM OVER_WARN R1-R27 R40-R57 R66-R89 TEMP_TRIM UNDER_CRIT UNDER_TRIM UNDER_WARN = rcl
BLINKER-L1 BLINKER-L2 BLINKER-R1 BLINKER-R2 BRAKE-C1 BRAKE-C2 BRAKE-L1 BRAKE-L2 BRAKE-R1 BRAKE-R2 OVERCURRENT_FET OVERTEMP1_FET OVERTEMP2_FET OVERVOLT_FET UNDERVOLT_FET = transistor-power
C7-C23 CONN1 IC6 L1 L2 PWR R28-R36 RX TX U$4 X1 = dp_devices
C56 C57 L5 L6 R39 = resistor
CONTACTOR IO OUTPUT POWER1 POWER3 VOLT = con-amp
D1 D2 = diode
IC5 = DP-EagleLibrary
IC7 = dp_devices; 93C46: 93C46
IC10 = microchip; MF: MICROCHIP; MPN: 24LC128-I/SNG; OC_FARNELL: 9757937; OC_NEWARK: 30H1511
JP1 JP2 = pinhead
JP3 JP4 = pinhead - Copy
JP7-JP15 = jumper
K1 = relay; MF: OMRON COMPONENTS USA; MPN: G2R-2-DC6; OC_FARNELL: unknown; OC_NEWARK: 89C5317
K2 = relay; MPN: G2R-2A-DC24; OC_FARNELL: 6985269; OC_NEWARK: 36M5257
K3 = relay; OC_FARNELL: unknown; OC_NEWARK: unknown
NEWBATT NEWBATT1-NEWBATT6 OLDBATT OLDBATT1-OLDBATT6 U$3 U$5 U$9 U$10 U$12-U$22 = SolarJackets_BMS
OVERCURRENT OVERTEMP1 OVERTEMP2 OVERVOLT OVERVOLT_WARN UNDERVOLT UNDERVOLT_WARN = led; MF: VISHAY SEMICONDUCTOR; OC_FARNELL: 1612435
POWER = con-phoenix-508; MPN: MSTBV 2,5/2-GF-5.08; OC_FARNELL: 1792792; OC_NEWARK: 69R9845
S1 = switch
SV1-SV4 = con-lstb; OC_FARNELL: unknown; OC_NEWARK: unknown
T1 T2 = zetex; OC_FARNELL: unknown; OC_NEWARK: unknown
U$2 U$11 = ADC_Research
X3 = con-coax; OC_FARNELL: unknown; OC_NEWARK: unknown

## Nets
1.8V: C9.+ C17.1 C18.1 C19.1 IC5.12 IC5.37 IC5.49 IC5.64 JP4.3
3.3V: 317CAP2.1 ADC1.16 ADC2.16 ADC3.16 ADC4.16 ADC_CAP1.1 ADC_CAP2.1 ADC_CAP3.1 ADC_CAP4.1 IC4.4 R21.1 U$6.16 U$7.16 U$8.8
3.3V1: 317CAP8.1 IC3.4 JP2.19 R19.1
3.3V2: 317CAP4.1 IC2.4 JP2.15 R11.1
3.3V3: C8.1 C10.1 C20.1 C21.1 C22.1 C23.1 IC5.20 IC5.31 IC5.42 IC5.50 IC5.56 IC6.2 IC7.6 IC7.8 JP3.1 JP4.2 L1.2 L2.2 PWR.A R30.1 R32.2 R33.2 R34.2 RX.A TX.A
3.3V4: 317CAP6.1 IC1.4 JP2.17 R13.1
3.3V+: IC10.2 IC10.8 R53.2 R54.2 U$3.1
5V: 3V2.1 6103CAP5.1 C2.1 PWR_1.2
5V1: C6.1 JP2.13 PWR_3.2
5V2: 3V.1 5V.2 6103CAP1.1 6484CAP1.1 7805CAP2.1 LMC6484_1.4
5V3: 3V1.1 6103CAP3.1 7805CAP3.1 IC13.2 SV3.2 SV3.5 SV3.8
5V4: 3V3.1 6103CAP7.1 JP2.9
5V5: 3V4.1 6103CAP9.1 C4.1 JP2.11 PWR_2.2
5V6: C7.1 CONN1.VUSB IC6.3 JP4.1
5V+: C45.2 C48.2 C49.2 C50.2 C54.2 C55.2 L6.1 U$2.P$13_ U$2.P$29_ U$11.8
12V: 5V.1 317CAP1.1 7805CAP1.1 IC4.3 SV2.1 U$1.8
12V1: K2.P1 POWER1.2 R24.2 R25.2
12V2: 7805CAP4.1 IC12.3 IC13.1 IC14.3 POWER3.2 R72.2 R73.2 R74.2 R75.2 R76.2 R77.2 R78.2 R79.2 R80.2 R81.2 R87.2 R88.2 R89.2
12V3: SV4.6 SV4.8 SV4.10 SV4.12 SV4.14 SV4.16 SV4.18 SV4.20
12V4: 317CAP3.1 317CAP5.1 317CAP7.1 C1.1 C3.1 C5.1 IC1.3 IC2.3 IC3.3 JP2.1 JP2.3 JP2.5 JP2.7 PWR_1.1 PWR_2.1 PWR_3.1
96V: R66.2 R67.2 R82.2 R83.2 VOLT.2
!PWEREN: IC5.60 JP3.3
!RESET: IC5.14 JP4.5 R30.2
!SUSPEND: IC5.36 JP4.22
A1: ADC1.1 LMC6484_1.1 LMC6484_1.2
A2: ADC1.2 LMC6484_1.6 LMC6484_1.7
A3: ADC1.3 LMC6484_1.8 LMC6484_1.9
A4: ADC1.4 LMC6484_1.13 LMC6484_1.14
AC0: IC5.26 JP4.14
AC1: IC5.27 JP4.15
AC2: IC5.28 JP4.16
AC3: IC5.29 JP4.17 R35.1
AC4: IC5.30 JP4.18 R36.1
AC5: IC5.32 JP4.19
AC6: IC5.33 JP4.20
AC7: IC5.34 JP4.21
AD0: IC5.16 JP4.6
AD1: IC5.17 JP4.7
AD2: IC5.18 JP4.8
AD3: IC5.19 JP4.9
AD4: IC5.21 JP4.10
AD5: IC5.22 JP4.11
AD6: IC5.23 JP4.12
AD7: IC5.24 JP4.13
AGND: 6484CAP1.2 ADC1.14 ADC2.14 ADC3.14 ADC4.14 LMC6484_1.11 R23.1 SV1.32 U$6.8 U$7.8 U$8.4
BC0: IC5.48 JP3.11
BC1: IC5.52 JP3.10
BC2: IC5.53 JP3.9
BC3: IC5.54 JP3.8
BC4: IC5.55 JP3.7
BC5: IC5.57 JP3.6
BC6: IC5.58 JP3.5
BC7: IC5.59 JP3.4
BD0: IC5.38 JP3.19
BD1: IC5.39 JP3.18
BD2: IC5.40 JP3.17
BD3: IC5.41 JP3.16
BD4: IC5.43 JP3.15
BD5: IC5.44 JP3.14
BD6: IC5.45 JP3.13
BD7: IC5.46 JP3.12
BLINKER_L: BLINKER-L1.1 BLINKER-L2.1 R5.2 R6.2 R10.2
BLINKER_L_BACK_-: BLINKER-L2.2 BLINKER-L2.4 SV4.13
BLINKER_L_FRONT_-: BLINKER-L1.2 BLINKER-L1.4 SV4.11
BLINKER_R: BLINKER-R1.1 BLINKER-R2.1 R7.1 R14.2 R15.2
BLINKER_R_BACK_-: BLINKER-R2.2 BLINKER-R2.4 SV4.17
BLINKER_R_FRONT_-: BLINKER-R1.2 BLINKER-R1.4 SV4.15
BRAKE: BRAKE-C1.1 BRAKE-L1.1 BRAKE-R1.1 R1.2 R3.2 R9.2 R16.2
BRAKE_C_-: BRAKE-C1.2 BRAKE-C1.4 BRAKE-C2.2 BRAKE-C2.4 SV4.7
BRAKE_L_-: BRAKE-L1.2 BRAKE-L1.4 BRAKE-L2.2 BRAKE-L2.4 SV4.9
BRAKE_R_-: BRAKE-R1.2 BRAKE-R1.4 BRAKE-R2.2 BRAKE-R2.4 SV4.5
BRAKE_REGEN: BRAKE-C2.1 BRAKE-L2.1 BRAKE-R2.1 R2.2 R4.2 R8.1 R17.2
CONTACTOR_IN: CONTACTOR.2 K3.S@
CONTACTOR_OUT: CONTACTOR.1 K3.P@
CURRENT: R84.2 SV3.7
D5V+: C51.2 C52.2 C53.2 L5.2 R51.2 R52.2 U$2.P$27_
DC+: POWER.1 S1.2
DGND0: C51.1 C52.1 C53.1 IC10.1 IC10.3 IC10.4 IC10.7 JP11.4 JP11.10 JP11.18 JP13.2 JP13.4 JP13.6 R53.1 U$2.P$28_
DIR: IO.2 R26.2
DM: CONN1.D- IC5.7
DP: CONN1.D+ IC5.8
EECLK: IC5.62 IC7.2 JP3.21 R32.1
EECS: IC5.63 IC7.1 JP3.20 R34.1
EEDATA: IC5.61 IC7.3 JP3.22 R31.2
GND: BLINKER-L1.3 BLINKER-L2.3 BLINKER-R1.3 BLINKER-R2.3 BRAKE-C1.3 BRAKE-C2.3 BRAKE-L1.3 BRAKE-L2.3 BRAKE-R1.3 BRAKE-R2.3 R1.1 R2.1 R3.1 R4.1 R5.1 R6.1 R14.1 R15.1 R16.1 R17.1 SV4.19
GND0: C45.1 C46.1 C47.1 C48.1 C49.1 C50.1 C54.1 C55.1 C56.2 C57.2 POWER.2 R56.2 R57.2 U$2.P$11_ U$2.P$12_ U$2.P$30_ U$11.4 X3.3 X3.4 X3.5
GND1: 3V2.3 3V3.3 3V4.3 317CAP3.2 317CAP4.2 317CAP5.2 317CAP6.2 317CAP7.2 317CAP8.2 6103CAP5.2 6103CAP6.2 6103CAP7.2 6103CAP8.2 6103CAP9.2 6103CAP10.2 C1.2 C2.2 C3.2 C4.2 C5.2 C6.2 JP1.2 JP1.4 JP1.6 JP1.8 JP1.10 JP1.12 JP1.14 JP1.16 JP1.18 JP1.20 JP1.22 JP1.24 JP1.26 JP1.28 JP1.30 JP1.32 JP1.34 JP1.36 JP1.38 JP1.40 JP1.42 JP1.44 JP1.46 JP1.48 JP1.50 JP1.52 JP1.54 JP1.56 JP1.58 JP1.60 JP2.2 JP2.4 JP2.6 JP2.8 JP2.10 JP2.12 JP2.14 JP2.16 JP2.18 JP2.20 PWR_1.3 PWR_2.3 PWR_3.3 R12.2 R18.2 R20.2
GND4: R57.1 U$3.2
GND5: 3V.3 5V.3 317CAP1.2 317CAP2.2 6103CAP1.2 6103CAP2.2 7805CAP1.2 7805CAP2.2 ADC1.9 ADC2.9 ADC3.9 ADC4.9 ADC_CAP1.2 ADC_CAP2.2 ADC_CAP3.2 ADC_CAP4.2 R22.2 R23.2 SV1.33 SV2.2 SV2.3 U$1.4
GND6: K2.P2 POWER1.1 T1.2 T2.2
GND7: C7.2 C8.2 C9.- C10.2 C11.2 C12.2 C13.- C14.- C15.2 C16.2 C17.2 C18.2 C19.2 C20.2 C21.2 C22.2 C23.2 CONN1.GND IC5.1 IC5.5 IC5.10 IC5.11 IC5.13 IC5.15 IC5.25 IC5.35 IC5.47 IC5.51 IC6.1 IC7.5 JP3.2 JP4.4 R28.1 R29.1
GND8: 3V1.3 6103CAP3.2 6103CAP4.2 7805CAP3.2 7805CAP4.2 CURRENT_TRIM.1 IC12.12 IC13.3 IC14.12 OVER_CRIT.1 OVER_TRIM.1 OVER_WARN.1 POWER3.1 SV3.3 SV3.6 SV3.9 TEMP_TRIM.1 UNDER_CRIT.1 UNDER_TRIM.1 UNDER_WARN.1 UNDERVOLT_FET.3 VOLT.1
IN1: LMC6484_1.3 SV1.1 U$6.1
IN2: LMC6484_1.5 SV1.2 U$6.2
IN3: LMC6484_1.10 SV1.3 U$6.3
IN4: LMC6484_1.12 SV1.4 U$6.4
IN5: ADC1.5 SV1.5 U$6.5
IN6: ADC1.6 SV1.6 U$6.6
IN7: ADC1.7 SV1.7 U$6.7
IN8: ADC1.8 SV1.8 U$6.9
IN9: ADC2.1 SV1.9 U$6.10
IN10: ADC2.2 SV1.10 U$6.11
IN11: ADC2.3 SV1.11 U$6.12
IN12: ADC2.4 SV1.12 U$6.13
IN13: ADC2.5 SV1.13 U$6.14
IN14: ADC2.6 SV1.14 U$6.15
IN15: ADC2.7 SV1.15 U$7.1
IN16: ADC2.8 SV1.16 U$7.2
IN17: ADC3.1 SV1.17 U$7.3
IN18: ADC3.2 SV1.18 U$7.4
IN19: ADC3.3 SV1.19 U$7.5
IN20: ADC3.4 SV1.20 U$7.6
IN21: ADC3.5 SV1.21 U$7.7
IN22: ADC3.6 SV1.22 U$7.9
IN23: ADC3.7 SV1.23 U$7.10
IN24: ADC3.8 SV1.24 U$7.11
IN25: ADC4.1 SV1.25 U$7.12
IN26: ADC4.2 SV1.26 U$7.13
IN27: ADC4.3 SV1.27 U$7.14
IN28: ADC4.4 SV1.28 U$7.15
IN29: ADC4.5 SV1.29 U$8.1
IN30: ADC4.6 SV1.30 U$8.2
IN31: ADC4.7 SV1.31 U$8.3
IN32: ADC4.8 U$1.1 U$8.5
MOTOR+: D2.C OUTPUT.2
MOTOR+_PRE: D2.A K1.O2 K1.S1
MOTOR-: D1.C OUTPUT.1
MOTOR-_PRE: D1.A K1.O1 K1.S2
N$1: R8.2 SV4.2
N$2: R7.2 SV4.4
N$3: R9.1 SV4.1
N$4: R10.1 SV4.3
N$5: IC2.1 R11.2 R12.1
N$6: IC1.1 R13.2 R18.1
N$7: IC3.1 R19.2 R20.1
N$8: IC4.1 R21.2 R22.1
N$9: K1.P2 K2.S1
N$10: K1.P1 K2.S2
N$11: K1.1 R24.1
N$12: K2.1 R25.1
N$13: K1.2 T1.1
N$14: K2.2 T2.1
N$15: R27.1 T2.3
N$16: R26.1 T1.3
N$17: IC5.6 R29.2
N$18: C11.1 IC5.2 X1.1
N$19: C12.1 IC5.3 X1.2
N$20: PWR.C R28.2
N$21: R35.2 RX.C
N$22: R36.2 TX.C
N$23: C41.1 R40.2 U$2.P$1_
N$24: C41.2 R41.2 U$2.P$2_
N$25: C42.1 R42.2 U$2.P$3_
N$26: C42.2 R43.2 U$2.P$4_
N$27: C43.1 R44.2 U$2.P$5_
N$28: C43.2 R45.2 U$2.P$6_
N$29: C44.1 R46.2 U$2.P$7_
N$30: C44.2 R47.2 U$2.P$8_
N$31: JP7.1 R40.1 R48.2 U$11.1
N$32: R48.1 U$11.2
N$33: JP7.3 U$11.3
N$34: JP8.1 R41.1 R49.2 U$11.7
N$35: R49.1 U$11.6
N$36: JP8.3 U$11.5
N$37: JP14.2 R42.1
N$38: JP14.1 R43.1
N$39: JP15.4 R44.1
N$40: JP15.3 R45.1
N$41: JP15.2 R46.1
N$42: JP15.1 R47.1
N$43: C46.2 JP9.2 U$2.P$9_
N$44: JP9.1 U$2.P$32_
N$45: IC7.4 R31.1 R33.1
N$46: JP10.2 U$2.P$31_
N$47: C47.2 JP10.1 U$2.P$10_
N$48: C14.+ C16.1 IC5.4 L2.1
N$49: C13.+ C15.1 IC5.9 L1.1
N$50: JP11.1 U$2.P$21_
N$51: R50.1 U$2.P$22_
N$52: JP11.3 JP11.5 R50.2
N$53: JP11.7 JP11.9 JP12.1 U$2.P$20_
N$54: JP11.11 U$2.P$18_
N$55: JP11.13 U$2.P$25_
N$56: JP11.15 U$2.P$23_
N$57: JP12.2 U$2.P$19_
N$58: JP11.17 JP12.3
N$59: JP13.1 U$2.P$16_
N$60: JP13.3 R51.1 U$2.P$17_
N$61: JP13.5 R52.1 U$2.P$24_
N$62: IC10.5 JP11.20
N$63: IC10.6 JP11.16
N$64: C57.1 IC15.2 L5.1 L6.2 R54.1 R55.1
N$65: IC15.1 R55.2 R56.1
N$66: C56.1 IC15.3 S1.1
N$74: NEWBATT.P$2 OLDBATT.P$2 U$5.P$1
N$75: NEWBATT.P$1 OLDBATT.P$1 U$9.P$1
N$78: NEWBATT1.P$2 OLDBATT1.P$2 U$10.P$1
N$79: NEWBATT1.P$1 OLDBATT1.P$1 U$12.P$1
N$82: NEWBATT2.P$2 OLDBATT2.P$2 U$13.P$1
N$83: NEWBATT2.P$1 OLDBATT2.P$1 U$14.P$1
N$86: NEWBATT3.P$2 OLDBATT3.P$2 U$15.P$1
N$87: NEWBATT3.P$1 OLDBATT3.P$1 U$16.P$1
N$90: NEWBATT4.P$2 OLDBATT4.P$2 U$17.P$1
N$91: NEWBATT4.P$1 OLDBATT4.P$1 U$18.P$1
N$94: NEWBATT5.P$2 OLDBATT5.P$2 U$19.P$1
N$95: NEWBATT5.P$1 OLDBATT5.P$1 U$20.P$1
N$98: NEWBATT6.P$2 OLDBATT6.P$2 U$21.P$1
N$99: NEWBATT6.P$1 OLDBATT6.P$1 U$22.P$1
N$169: IC12.7 UNDER_WARN.2
N$170: IC12.5 UNDER_CRIT.2
N$171: IC12.9 IC12.11 TEMP_TRIM.2
N$172: R66.1 UNDER_CRIT.3
N$173: R67.1 UNDER_WARN.3
N$174: IC12.4 IC12.6 UNDER_TRIM.2
N$175: R71.1 UNDER_TRIM.3
N$176: R70.1 TEMP_TRIM.3
N$177: R72.1 UNDERVOLT.A
N$178: R73.1 UNDERVOLT_WARN.A
N$179: OVERTEMP1.A R74.1
N$180: OVERTEMP2.A R75.1
N$181: K3.1 R77.1
N$182: CURRENT_TRIM.2 IC14.9
N$183: OVER_WARN.3 R83.1
N$184: IC14.5 IC14.7 OVER_TRIM.2
N$185: OVER_TRIM.3 R86.1
N$186: CURRENT_TRIM.3 R85.1
N$187: OVERVOLT.A R87.1
N$188: OVERVOLT_WARN.A R88.1
N$189: OVERCURRENT.A R89.1
N$190: K3.2 OVERCURRENT_FET.2 OVERCURRENT_FET.4
N$191: OVERCURRENT_FET.3 OVERTEMP2_FET.2 OVERTEMP2_FET.4
N$192: OVERTEMP1_FET.2 OVERTEMP1_FET.4 OVERTEMP2_FET.3
N$193: OVERTEMP1_FET.3 OVERVOLT_FET.2 OVERVOLT_FET.4
N$194: OVERVOLT_FET.3 UNDERVOLT_FET.2 UNDERVOLT_FET.4
N$195: IC14.6 OVER_WARN.2
N$196: IC14.4 OVER_CRIT.2
N$197: OVER_CRIT.3 R82.1
N$198: IC14.8 R84.1
N$199: IC12.8 R68.1
N$200: IC12.10 R69.1
ON: IO.1 R27.2
OVERCURRENT_CRITICAL: IC14.14 OVERCURRENT.K OVERCURRENT_FET.1 R81.1
OVERTEMP_CRITICAL1: IC12.14 OVERTEMP1.K OVERTEMP1_FET.1 R79.1
OVERTEMP_CRITICAL2: IC12.13 OVERTEMP2.K OVERTEMP2_FET.1 R80.1
OVERVOLT_CRITICAL: IC14.2 OVERVOLT.K OVERVOLT_FET.1 R78.1
OVERVOLT_WARNING1: IC14.1 OVERVOLT_WARN.K
SIGNALGND: JP8.2 JP14.3 R39.2 X3.2
SIGNALV+: JP7.2 JP14.4 R39.1 X3.1
SPI_CLK: ADC1.13 ADC2.13 ADC3.13 ADC4.13 SV2.10
SPI_CS1: ADC1.10 SV2.7
SPI_CS2: ADC2.10 SV2.6
SPI_CS3: ADC3.10 SV2.5
SPI_CS4: ADC4.10 SV2.4
SPI_DIN: ADC1.11 ADC2.11 ADC3.11 ADC4.11 SV2.8
SPI_DOUT: ADC1.12 ADC2.12 ADC3.12 ADC4.12 SV2.9
TEMP1: R68.2 SV3.1
TEMP2: R69.2 SV3.4
UNDERVOLT_CRITICAL: IC12.2 R76.1 UNDERVOLT.K UNDERVOLT_FET.1
UNDERVOLT_WARNING: IC12.1 UNDERVOLT_WARN.K
VREF: 3V.2 6103CAP2.1 ADC1.15 ADC2.15 ADC3.15 ADC4.15 SV1.34
VREF1: 3V1.2 6103CAP4.1 R70.2 R71.2 R85.2 R86.2
VREF2: 3V2.2 6103CAP6.1 JP1.1 JP1.3 JP1.5 JP1.7 JP1.9 JP1.11 JP1.13 JP1.15 JP1.17 JP1.19
VREF3: 3V3.2 6103CAP8.1 JP1.21 JP1.23 JP1.25 JP1.27 JP1.29 JP1.31 JP1.33 JP1.35 JP1.37 JP1.39
VREF4: 3V4.2 6103CAP10.1 JP1.41 JP1.43 JP1.45 JP1.47 JP1.49 JP1.51 JP1.53 JP1.55 JP1.57 JP1.59

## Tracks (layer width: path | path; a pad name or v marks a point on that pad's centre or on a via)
1.8V  (via drill 0.38)
  Top 0.254: C19.1 188.98,30.1 190.75,31.88 190.75,32.69 | 198.09,32.64 IC5.12 198.09,27.14 C17.1 | 198.09,32.64 198.09,38.45 v198.12,38.73 | v198.12,40.51 198.09,40.54 IC5.37 198.09,44.17 200.15,46.23 C18.1 | v192.79,40.51 192.47,40.2 IC5.49 187.87,40.2 C9.+ | 190.75,32.69 198.04,32.69 198.09,32.64 | 190.75,32.69 IC5.64
  Top 0.305: C17.1 199.33,26.73 200.03,26.04 200.03,23.75 200.79,22.99 203.33,22.99 v207.65,18.67
  Bottom 0.254: v198.12,38.73 v198.12,40.51 v192.79,40.51
  Bottom 0.305: v207.65,18.67 210.19,16.13 210.19,9.27 JP4.3
3.3V  (via drill 0.38)
  Top 0.254: ADC_CAP1.1 105.66,46.23 105.66,42.88 106.93,41.6 ADC1.16 106.98,41.48 106.98,40.23 109.17,38.05 120.24,38.05 | U$6.16 124.08,31.34 120.24,35.18 120.24,38.05 | 120.24,38.05 120.24,40.87 120.85,41.48 ADC2.16 120.9,42.19 121.74,43.03 122.15,43.03 ADC_CAP2.1 125.48,46.28 v127.53,48.34 | U$7.16 138.05,27.51 138.86,26.7 150.6,26.7 152.02,28.12 U$8.8 151.97,28.25 151.97,30.38 148.16,34.19 148.16,39.9 148.79,40.54 148.79,41.48 ADC4.16 148.84,42.39 150.34,43.89 ADC_CAP4.1 150.24,46.3 140.59,46.3 139.7,47.19 | 142.37,57.99 317CAP2.1 | 142.37,57.99 143.76,56.59 IC4.4 | 139.93,55.58 138.43,55.58 R21.1 | 139.93,55.58 142.26,57.91 142.37,57.99 | ADC3.16 134.87,42.57 137.39,45.09 ADC_CAP3.1 137.49,46.81 138.2,47.52 139.37,47.52 139.7,47.19 | v140,52.86 140,55.47 139.93,55.58 | 139.7,47.19 v140,47.5
  Bottom 0.254: v140,47.5 140,48.34 | 140,48.34 v140,52.86 | 140,48.34 v127.53,48.34
3.3V1
  Top 0.254: 91.82,24.77 86.74,29.84 317CAP8.1 | 91.82,24.77 95.25,28.19 96.9,28.19 R19.1 | 91.82,24.77 IC3.4 91.69,24.77 91.69,17.02 77.98,3.3 38.35,3.3 37.34,4.32 37.34,5.84 JP2.19
3.3V2  (via drill 0.61)
  Top 0.254: 14.35,32.51 10.79,36.07 9.27,36.07 IC2.4 9.27,36.2 5.84,32.77 4.19,32.77 R11.1 | 14.35,32.51 v15.88,32.51 | 14.35,32.51 317CAP4.1
  Bottom 0.254: JP2.15 37.08,14.73 30.35,14.73 28.83,16.26 28.83,19.56 v15.88,32.51
3.3V3  (via drill 0.38, 0.51)
  Top 0.254: C22.1 196.34,47.12 195.59,46.37 IC5.42 195.59,39.71 195.58,39.7 | 199.64,39.7 IC5.31 203.78,39.7 204.47,40.39 C21.1 | 195.58,39.7 199.64,39.7 | 195.58,39.7 IC5.50 189.56,39.7 188.85,38.99 188.85,36.7 | 199.64,39.7 199.64,35.18 200.62,34.2 IC5.20 204.81,34.2 205.55,33.46 C20.1 | 188.85,36.7 IC5.56 | 188.85,36.7 C23.1
  Top 0.305: C10.1 184.34,51.82 IC7.8 188.98,51.82 189.1,51.94 | C22.1 190.31,48.2 189.1,49.4 189.1,51.94 | R34.2 R33.2 198.5,56.77 198.25,57.02 189.87,57.02 189.1,56.26 189.1,54.48 | R34.2 R32.2 | 189.1,51.94 189.1,54.48 | IC7.6 188.98,54.36 189.1,54.48 | R34.2 206.35,55.81 TX.A RX.A | R30.1 203.27,24.96 v203.33,25.02
  Top 0.406: 205.87,12.57 IC6.2 205.87,8.26 208.79,5.33 JP4.2 | 205.87,12.57 205.87,15.88 v206.63,16.64 204.69,18.58 L1.2 | C8.1 205.93,12.64 205.87,12.57 | C23.1 187.13,35.49 183.51,31.88 183.51,13.34 | 183.51,2.79 185.26,2.79 PWR.A 188.94,2.76 v189.1,2.92 | 183.51,2.79 JP3.1 | 183.51,2.79 183.51,13.34 | L2.2 183.6,13.25 183.51,13.34 | C20.1 205.55,29.14 v206.63,28.07
  Bottom 0.305: 206.63,25.02 v203.33,25.02
  Bottom 0.406: v206.63,16.64 206.63,25.02 v206.63,28.07 | v189.1,2.92 209.17,2.92 JP4.2
3.3V4  (via drill 0.61)
  Top 0.254: 75.31,45.09 80.39,40.01 317CAP6.1 | 75.31,45.09 71.88,41.66 70.23,41.66 R13.1 70.23,41.53 69.47,41.53 v58.8,30.86 | 75.31,45.09 IC1.4 | v49.4,15.37 JP2.17
  Bottom 0.254: v49.4,15.37 49.4,21.46 v58.8,30.86
3.3V+  (via drill 0.61)
  Top 0.254: 229.95,94.69 229.95,97.16 | 229.95,97.16 229.95,98.42 R53.2 | 229.95,94.69 229.74,94.69 IC10.2 | IC10.8 230.38,90.12 230.38,94.61 230.05,94.61 229.95,94.69 | 209.59,111.77 201.88,104.06 201.88,98.7 203.25,98.7 204.8,97.16 R54.2 | 209.59,111.77 214.17,116.36 U$3.1 | v230.07,101.58 229.69,101.19 220.17,101.19 209.59,111.77 | v230.05,97.16 229.95,97.16
  Bottom 0.254: v230.05,97.16 230.07,97.18 v230.07,101.58
5V
  Top 0.254: 3V2.1 75.56,28.19 75.31,28.45 72.77,28.45 6103CAP5.1 72.77,28.57 59.82,28.57 55.75,32.64 36.45,32.64 30.67,38.42 | 30.67,38.42 26.8,34.54 PWR_1.2 | 30.67,38.42 30.86,38.61 C2.1
5V1  (via drill 0.61)
  Top 0.254: C6.1 63.88,38.61 59.82,34.54 PWR_3.2 59.69,34.54 v59.69,33.02 | v54.48,15.37 JP2.13
  Bottom 0.254: v54.48,15.37 54.48,25.27 59.69,30.48 v59.69,33.02
5V2  (via drill 0.38)
  Top 0.254: v115.88,25.07 116.43,24.51 6484CAP1.1 | v110.92,24.89 112.01,23.8 LMC6484_1.4 | 128.5,57.53 128.5,56.13 128.07,55.7 3V.1 | 128.5,57.53 128.5,58.55 6103CAP1.1 | 113.41,52.45 114.1,52.45 114.33,52.22 5V.2 | 113.41,52.45 7805CAP2.1 109.93,52.35 v108.58,51 | 128.5,57.53 118.39,57.53 113.41,52.55 113.41,52.45
  Bottom 0.254: 108.51,32.44 v115.88,25.07 | 108.51,32.44 107.9,32.44 107.47,32 107.47,28.35 v110.92,24.89 | v108.58,51 108.58,32.54 108.51,32.44
5V3
  Top 0.254: SV3.5 SV3.8 71.4,66.09 69.83,67.67 | SV3.2 64.19,66.04 65.81,67.67 69.83,67.67 | 37.47,122.53 38.38,122.53 38.79,122.12 3V1.1 | 37.47,122.53 6103CAP3.1 | 37.47,122.53 37.47,124.41 38.89,125.83 54.18,125.83 58.29,121.72 60.12,121.72 62.26,119.58 IC13.2 62.36,119.63 65.25,122.53 7805CAP3.1 67.79,122.48 68.15,122.48 71.3,119.33 71.3,104.19 70.94,103.83 70.94,95.96 71.14,95.76 71.14,89.92 71.3,89.76 71.3,78.79 69.88,77.37 69.88,67.77 69.83,67.67
5V4  (via drill 0.61)
  Top 0.254: 6103CAP7.1 48.64,28.45 51.18,28.45 51.44,28.19 3V3.1 51.56,28.07 v51.56,20.19
  Bottom 0.254: v51.56,20.19 51.56,19.68 51.69,19.56 51.69,7.75 JP2.9
5V5  (via drill 0.61)
  Top 0.254: 6103CAP9.1 23.24,28.45 v24.77,28.45 25.78,28.45 26.04,28.19 3V4.1 | C4.1 47.37,38.61 43.31,34.54 PWR_2.2 43.18,34.67 v42.04,33.53
  Bottom 0.254: v24.77,28.45 36.96,28.45 37.02,28.51 | v42.04,33.53 37.02,28.51 | JP2.11 49.28,8.51 41.53,16.26 41.53,24 37.02,28.51
5V6  (via drill 0.38, 0.51)
  Top 0.305: v203.58,6.99 203.57,7
  Top 0.406: C7.1 204.34,11.68 203.57,10.91 IC6.3 203.57,7 | CONN1.VUSB 194.74,7.7 v195.71,6.73 | v203.58,6.99 206.12,6.99 210.31,2.79 JP4.1
  Bottom 0.406: v195.71,6.73 197.23,5.21 201.8,5.21 v203.58,6.99
5V+  (via drill 0.61)
  Top 0.254: 235.79,106.02 235.79,107.16 236.07,107.16 236.27,107.37 236.27,107.92 U$2.P$29_ | 235.79,106.02 235.79,103 U$2.P$13_ 235.76,102.87 235.76,102.41 234.9,101.55 233.88,101.55 233.07,100.74 224.33,100.74 v219.53,95.94 | v235.89,106.02 235.79,106.02 | v239.29,101.73 v246.15,101.73
  Bottom 0.254: L6.1 216.15,88.27 216.26,88.37 216.26,91.69 C54.2 216.64,92.18 C55.2 216.76,95.94 v219.53,95.94 | C45.2 246.89,110.11 248.08,110.11 248.08,109.96 249.86,108.18 249.86,107.95 U$11.8 249.83,107.82 249.71,107.7 249.71,105.79 246.15,102.23 v246.15,101.73 | C49.2 C50.2 238.1,112.55 238.86,112.55 238.86,111.89 239.95,110.8 239.95,108.48 237.58,106.11 | C48.2 232.92,110.11 234.11,108.92 234.11,108.74 235.89,106.96 v235.89,106.02 235.99,105.94 237.41,105.94 237.58,106.11 | v239.29,101.73 239.52,101.96 239.52,104.17 237.58,106.11
12V  (via drill 0.38)
  Top 0.254: 7805CAP1.1 113.84,56.26 114.33,56.74 5V.1 114.45,56.79 116.71,56.79 120.7,60.78 146.07,60.78 146.33,60.53 317CAP1.1 146.43,60.45 147.45,60.45 | 147.45,60.45 155.27,60.45 158.37,57.35 U$1.8 158.42,57.23 158.42,56.67 159.18,55.91 164.47,55.91 174.07,46.3 174.07,37.77 172.97,36.68 SV2.1 | v146.07,52.3 IC4.3 | 147.45,60.45 v147.45,59.82
  Bottom 0.254: v146.07,52.3 146.07,58.45 v147.45,59.82
12V1
  Top 0.254: R24.2 164.68,112.27 164.68,100.2 POWER1.2 | 163.03,98.93 163.03,90.3 166.21,90.3 169.63,93.73 169.63,110.87 171.03,112.27 R25.2
  Top 2.794: POWER1.2 163.03,98.93 150.08,98.93 150.08,111 137.05,111 K2.P1
12V2  (via drill 0.38)
  Top 0.254: IC12.3 62.66,88.9 63.78,90.02 63.78,105.56 62.66,106.68 IC14.3 61.29,106.73 60.07,106.73 58.7,108.1 58.7,111.86 53.34,117.22 | v54.63,122.53 7805CAP4.1 | IC13.1 57.78,119.69 57.48,119.69 v56.67,120.5 56.57,120.45 53.34,117.22 | 35.13,114.3 R77.2 43.26,114.25 45.03,116.03 52.15,116.03 53.34,117.22 | 35.13,114.3 33.86,115.57 R76.2 | R73.2 12.22,118.11 12.22,111.86 R88.2 12.22,111.76 12.22,105.51 R72.2 12.22,105.41 12.22,99.16 R87.2 12.22,99.06 12.22,92.81 R74.2 12.22,92.71 12.22,86.46 R75.2 12.22,86.36 12.22,80.01 R89.2 12.32,79.91 21.26,79.91 22.89,78.28 31.42,78.28 33.71,80.57 R81.2 | R81.2 33.81,80.01 33.81,88.9 R80.2 33.81,89 33.81,97.79 R79.2 33.81,97.89 33.81,106.68 R78.2 33.86,106.78 33.86,110.85 35.08,112.06 35.08,114.2 35.13,114.3 | POWER3.2 37.21,76.5 33.81,79.91 R81.2
  Bottom 0.254: v56.67,120.5 v54.63,122.53
12V3
  Top 0.254: SV4.20 SV4.18 SV4.16 SV4.14 SV4.12 SV4.10 SV4.8 SV4.6
12V4  (via drill 0.61)
  Top 0.254: 317CAP7.1 92.46,34.29 92.46,33.91 v91.44,32.89 89.53,30.99 IC3.3 | 317CAP5.1 74.68,35.56 74.68,35.94 v75.69,36.96 77.6,38.86 IC1.3 | 317CAP3.1 8.64,26.67 8.64,27.05 v9.65,28.07 11.56,29.97 IC2.3 | v19.43,41.15 C1.1 | v35.94,41.15 C3.1 | v52.45,41.15 C5.1 | v23.5,34.67 22.35,34.67 PWR_1.1 | v40.01,34.67 38.86,34.67 PWR_2.1 | v56.52,34.67 55.37,34.67 PWR_3.1
  pour Bottom: 1.65,1.27 99.44,1.27 99.44,50.8 1.65,50.8
96V  (via drill 0.38)
  Top 0.254: 86.33,80.01 R83.2 86.23,80.62 | 86.33,92.71 R67.2 86.33,92.81 | 86.33,105.41 R82.2 86.33,105.51 | 86.33,118.11 R66.2
  Top 0.61: 86.33,92.71 86.33,80.01 | 86.33,92.81 86.33,105.41 | 86.33,105.51 86.33,118.11 | v71.7,76.1 81.71,76.1 86.23,80.62
  Bottom 0.254: 21.97,70.46 VOLT.2
  Bottom 0.61: 21.97,70.46 27,70.46 36.09,61.37 56.97,61.37 v71.7,76.1
!PWEREN  (via drill 0.38)
  Top 0.254: IC5.60 189.89,34.7 189.61,34.42 v189.61,32.13
  Bottom 0.254: v189.61,32.13 187.07,29.59 187.07,13.08 JP3.3
!RESET
  Top 0.254: JP4.5 208.91,15.62 208.91,20.95 203.01,26.86 R30.2 201.68,28.7 201.04,29.34 199.77,29.34 199.09,30.02 IC5.14
!SUSPEND  (via drill 0.38)
  Top 0.254: IC5.36 198.59,43.91 v204.34,49.66
  Bottom 0.254: v204.34,49.66 205.1,49.66 JP4.22
A1
  Top 0.254: LMC6484_1.2 LMC6484_1.1 108.13,23.29 106.93,24.49 ADC1.1
A2  (via drill 0.38)
  Top 0.254: LMC6484_1.7 LMC6484_1.6 114.83,23.29 v114.83,25.07 | v108.2,31.7 ADC1.2
  Bottom 0.254: v114.83,25.07 v108.2,31.7
A3  (via drill 0.38)
  Top 0.254: 115.04,28.4 115.82,28.4 LMC6484_1.8 | 115.04,28.4 114.55,28.4 LMC6484_1.9 | v109.47,34.06 ADC1.3 | v113.44,30.1 115.04,28.5 115.04,28.4
  Bottom 0.254: v113.44,30.1 v109.47,34.06
A4
  Top 0.254: 108.99,28.4 109.47,28.4 LMC6484_1.13 | 108.99,28.4 108.2,28.4 LMC6484_1.14 | ADC1.4 110.74,30.25 108.99,28.5 108.99,28.4
AC0
  Top 0.254: IC5.26 208.93,37.2 210.31,35.81 JP4.14
AC1
  Top 0.254: IC5.27 209.15,37.7 209.8,38.35 JP4.15
AC2
  Top 0.254: IC5.28 208.89,38.2 JP4.16
AC3
  Top 0.254: IC5.29 208.62,38.7 209.93,40.01 209.93,41.78 JP4.17 212.98,44.83 212.98,46.61 212.34,47.24 210.95,47.24 209.99,48.2 R35.1
AC4
  Top 0.254: R36.1 206.38,46.86 207.26,45.97 209.42,45.97 | 209.42,45.97 JP4.18 | 209.42,45.97 209.42,40.26 208.36,39.2 IC5.30
AC5  (via drill 0.38)
  Top 0.254: IC5.32 203.01,40.2 v205.1,42.29
  Bottom 0.254: v205.1,42.29 205.36,42.29 JP4.19
AC6  (via drill 0.38)
  Top 0.254: IC5.33 202.58,42.05 v204.34,43.81
  Bottom 0.254: JP4.20 v204.34,43.81
AC7  (via drill 0.38)
  Top 0.254: IC5.34 199.59,42.87 v204.34,47.62
  Bottom 0.254: v204.34,47.62 205.61,47.62 JP4.21
AD0
  Top 0.254: IC5.16 201.31,30.85 202.82,29.34 202.82,27.81 209.42,21.21 209.42,17.65 JP4.6
AD1
  Top 0.254: IC5.17 203.01,32.7 203.33,32.38 203.33,28.07 209.93,21.46 209.93,19.68 JP4.7
AD2
  Top 0.254: IC5.18 203.28,33.2 203.84,32.64 203.84,28.32 JP4.8
AD3
  Top 0.254: IC5.19 203.54,33.7 204.34,32.89 204.34,28.57 209.8,23.11 JP4.9
AD4
  Top 0.254: IC5.21 206.85,34.7 209.17,32.38 209.17,28.07 JP4.10
AD5
  Top 0.254: IC5.22 207.12,35.2 209.68,32.64 209.68,30.1 JP4.11
AD6
  Top 0.254: IC5.23 207.38,35.7 210.19,32.89 210.19,32.13 JP4.12
AD7
  Top 0.254: IC5.24 207.64,36.2 210.57,33.27 JP4.13
AGND  (via drill 0.38)
  Top 0.254: R23.1 157.78,24.89 U$8.4 155.88,22.81 155.88,22.05 157.66,20.27 157.66,11.02 SV1.32 156.64,9.83 154.74,9.83 154.1,10.46 154.1,11.02 146.94,18.19 U$7.8 146.89,23.04 146.89,23.6 145.11,25.38 137.08,25.38 v134.39,22.68 | v109.47,38.79 ADC1.14 | v111.96,32.61 111.96,28.5 LMC6484_1.11 112.01,27.76 113.97,25.81 6484CAP1.2 119.05,25.68 130.84,25.68 132.97,23.55 U$6.8 132.92,22.81 v132.92,21.21 | ADC2.14 123.44,40.95 v122.38,39.88 | v130.43,39.98 136.42,39.98 137.41,40.97 ADC3.14 137.47,41.71 137.47,43.61 137.9,44.04 138.51,44.04 v139.32,43.23 | ADC4.14 151.38,42.57 v150.72,43.23
  Bottom 0.254: v111.96,32.61 109.47,35.1 v109.47,38.79 109.58,38.86 110.59,39.88 v122.38,39.88 122.48,39.8 123.14,39.14 123.75,39.14 124.59,39.98 v130.43,39.98 | v139.32,43.23 v150.72,43.23 | v132.92,21.21 v134.39,22.68
  other vias: 123.44,17.91 122.17,13.08 115.19,16.64 119.63,33.78 132.97,36.96
  pour Top: 103.12,39.5 164.72,39.5 164.72,1.4 103.12,1.4
  pour Bottom: 103.12,39.5 164.72,39.5 164.72,1.4 103.12,1.4
BC0  (via drill 0.38)
  Top 0.254: IC5.48 191.66,42.05 v191.64,42.04
  Bottom 0.254: v191.64,42.04 183.01,33.4 183.01,30.1 JP3.11
BC1  (via drill 0.38)
  Top 0.254: IC5.52 194.22,38.7 v194.69,38.23
  Bottom 0.254: v194.69,38.23 188.59,38.23 183.51,33.15 183.51,28.07 JP3.10
BC2  (via drill 0.38)
  Top 0.254: IC5.53 192.94,38.2 v193.93,37.21
  Bottom 0.254: v193.93,37.21 188.34,37.21 184.02,32.89 184.02,26.04 JP3.9
BC3  (via drill 0.38)
  Top 0.254: IC5.54 192.17,37.7 192.91,36.96 v192.91,36.2
  Bottom 0.254: v192.91,36.2 188.09,36.2 184.53,32.64 184.53,24 JP3.8
BC4  (via drill 0.38)
  Top 0.254: IC5.55 191.66,37.2 191.9,36.96 v191.9,35.18
  Bottom 0.254: v191.9,35.18 187.83,35.18 185.04,32.38 185.04,21.97 JP3.7
BC5  (via drill 0.38)
  Top 0.254: IC5.57 189.11,36.2 186.06,33.15 v186.06,32.13
  Bottom 0.254: JP3.6 185.55,19.94 185.55,31.62 v186.06,32.13
BC6  (via drill 0.38)
  Top 0.254: IC5.58 189.37,35.7 187.58,33.91 v187.58,33.4
  Bottom 0.254: v187.58,33.4 187.58,32.38 186.06,30.86 186.06,17.91 JP3.5
BC7  (via drill 0.38)
  Top 0.254: IC5.59 189.63,35.2 188.59,34.16 v188.59,32.77
  Bottom 0.254: v188.59,32.77 188.59,32.64 186.56,30.61 186.56,15.11 JP3.4
BD0  (via drill 0.38)
  Top 0.254: IC5.38 197.59,44.43 199.01,45.85 199.01,48.13 v198.25,48.9
  Bottom 0.254: v198.25,48.9 197.23,49.91 191.39,49.91 189.99,48.51 JP3.19
BD1  (via drill 0.38)
  Top 0.254: IC5.39 197.09,44.69 198.5,46.1 198.5,47.12 v197.99,47.62
  Bottom 0.254: v197.99,47.62 196.22,49.4 191.64,49.4 188.21,45.97 JP3.18
BD2  (via drill 0.38)
  Top 0.254: IC5.40 196.59,44.95 197.49,45.85 v197.49,46.61
  Bottom 0.254: v197.49,46.61 195.2,48.9 191.9,48.9 186.44,43.43 JP3.17
BD3  (via drill 0.38)
  Top 0.254: IC5.41 196.09,45.72 v196.47,46.1
  Bottom 0.254: v196.47,46.1 196.47,46.86 194.94,48.39 192.15,48.39 184.66,40.89 JP3.16
BD4  (via drill 0.38)
  Top 0.254: IC5.43 195.09,46.97 v194.69,47.37
  Bottom 0.254: v194.69,47.37 191.9,47.37 182.88,38.35 JP3.15
BD5  (via drill 0.38)
  Top 0.254: IC5.44 194.59,45.95 v194.18,46.35
  Bottom 0.254: v194.18,46.35 191.64,46.35 JP3.14
BD6  (via drill 0.38)
  Top 0.254: IC5.45 194.09,44.92 v193.68,45.34
  Bottom 0.254: v193.68,45.34 192.15,45.34 190.12,43.31 190.12,42.04 181.48,33.4 181.1,33.4 JP3.13
BD7  (via drill 0.38)
  Top 0.254: IC5.46 193.59,43.64 v192.91,44.32
  Bottom 0.254: v192.91,44.32 191.9,44.32 190.63,43.05 190.63,41.78 182.5,33.66 182.5,32.13 JP3.12
BLINKER_L  (via drill 0.38, 0.61)
  Top 0.254: 234.19,25.65 236.09,25.65 R6.2 | 234.19,25.65 232.28,25.65 R5.2 | v248.92,25.78 251.33,25.78 R10.2 | v247.65,27.05 247.01,27.69 234.31,27.69 | 224.16,27.69 234.31,27.69 | 224.16,27.69 221.11,30.73 BLINKER-L2.1 221.11,30.86 | v234.19,26.29 234.19,25.65 | 234.31,27.69 v234.31,28.07 | 221.11,40.89 BLINKER-L1.1 | 224.16,27.69 224.16,27.81 v223.39,28.57
  Top 0.406: 221.11,40.89 221.11,37.72 v220.85,37.72
  Bottom 0.254: v247.65,27.05 v248.92,25.78 | v234.19,26.29 234.31,26.42 v234.31,28.07
  Bottom 0.406: v220.85,37.72 220.85,29.27 222.69,29.27 v223.39,28.57
BLINKER_L_BACK_-  (via drill 0.61)
  Top 0.254: BLINKER-L2.4 BLINKER-L2.2 223.39,30.73 v225.55,28.57 | SV4.13 245.11,9.91 230.5,9.91 229.87,10.54 v229.87,23.5
  Bottom 0.254: v229.87,23.5 225.55,27.81 v225.55,28.57
  pour Top: 227.2,37.72 227.2,2.16 215.77,2.16 215.77,37.72
BLINKER_L_FRONT_-  (via drill 0.38)
  Top 0.254: BLINKER-L1.4 223.39,42.42 | 223.39,42.42 BLINKER-L1.2 | 223.39,42.42 v218.69,42.42
  Bottom 0.254: SV4.11 244.86,12.19 246.76,12.19 247.4,11.56 247.4,9.4 230.25,9.4 218.69,20.95 v218.69,42.42
  pour Top: 227.2,38.99 227.2,61.85 215.77,61.85 215.77,38.99
BLINKER_R  (via drill 0.61)
  Top 0.254: BLINKER-R1.1 256.67,40.89 256.67,30.86 BLINKER-R2.1 256.67,30.73 v256.67,28.07 | 256.67,25.65 258.95,25.65 R15.2 | 256.67,25.65 255.14,25.65 | 255.14,25.65 251.97,22.48 241.68,22.48 239.9,24.26 R7.1 | 255.14,25.65 R14.2 | 256.67,25.65 v256.67,25.78
  Bottom 0.254: v256.67,25.78 v256.67,28.07
BLINKER_R_BACK_-
  Top 0.254: BLINKER-R2.4 BLINKER-R2.2 258.95,30.73 260.35,29.34 267.46,29.34 267.46,23.88 256.03,12.45 252.73,12.45 SV4.17
  pour Top: 255.14,2.16 255.14,37.72 267.84,37.72 267.84,2.16
BLINKER_R_FRONT_-  (via drill 0.61)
